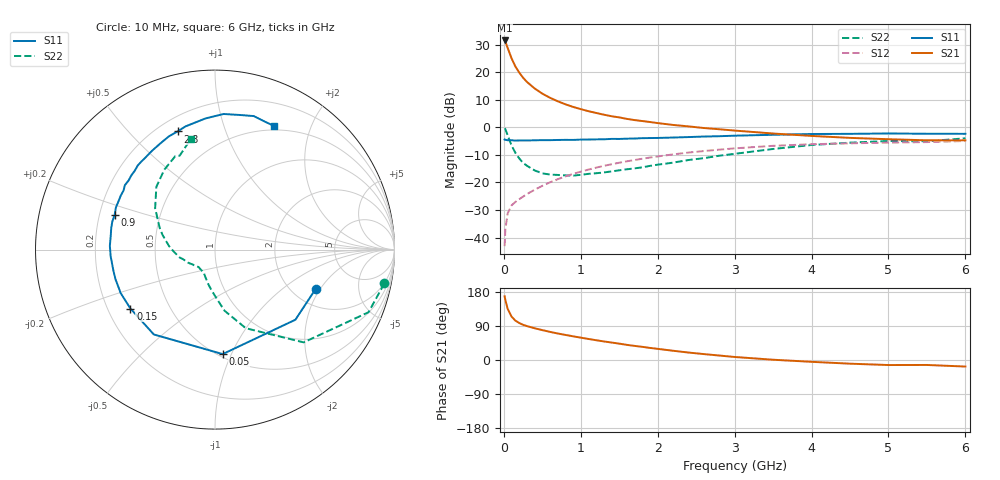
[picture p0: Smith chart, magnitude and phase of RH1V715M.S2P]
! SIEMENS Small Signal Semiconductors
! BFR106
! Si NPN RF Bipolar Junction Transistor in SOT23
! VCE = 1.75 V  IC = 15 mA
! Common Emitter S-Parameters:  August  1996
# GHz  S  MA  R  50
!  f  S11  S21  S12  S22
! GHz  MAG  ANG  MAG  ANG  MAG  ANG  MAG  ANG
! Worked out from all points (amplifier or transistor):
!   36 points, 10 MHz to 6 GHz, reference 50 ohm
!   highest |S21| = 31.5 dB at 10 MHz (marker M1)
!   |S21| within 3 dB of that: start of sweep to 53.49 MHz
!   unconditionally stable (mu >= 1): 393.3 MHz to 2.511 GHz; 4.668 GHz to end of sweep
!   at 250 MHz: K = 0.84, MSG = 21.6 dB, |S12| = -25.1 dB
!   at 1.4 GHz: K = 1.09, MAG = 6.9 dB, |S12| = -13.4 dB
!   at 6 GHz: K = 1.02, MAG = -0.8 dB, |S12| = -5.0 dB
!   S11 on the Smith chart (normalised r, x): 10 MHz: 2.65, -1.82; 50 MHz: 0.53, -0.93; 150 MHz: 0.29, -0.29; 900 MHz: 0.26, +0.16; 2.8 GHz: 0.28, +0.69; 6 GHz: 0.45, +1.49
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0.01  0.6023 -21.3  37.64 168.2  0.007 82.6  0.9624 -11.3
0.02  0.5944 -41.1  35.84 158.2  0.0143 74.7  0.9237 -22.2
0.05  0.5837 -85.8  27.46 134.7  0.0276 57.1  0.7149 -46.3
0.1  0.5829 -125.8  17.88 114.6  0.0384 48.1  0.4704 -68.6
0.15  0.5743 -145.1  12.7 103.9  0.0444 47.1  0.3449 -81.1
0.2  0.5787 -155.2  9.844 97.7  0.0497 49.0  0.2734 -88.0
0.25  0.5784 -163.2  7.937 92.8  0.0555 51.0  0.2265 -95.0
0.3  0.5781 -168.0  6.672 89.5  0.0616 53.8  0.2014 -99.9
0.4  0.5825 -176.3  5.076 83.8  0.0737 57.2  0.1657 -108.3
0.5  0.5862 178.0  4.086 78.9  0.0869 59.1  0.1465 -114.6
0.6  0.5857 172.9  3.437 74.2  0.1007 60.3  0.1392 -119.8
0.7  0.5903 168.4  2.973 70.0  0.1146 61.1  0.1371 -124.8
0.9  0.5915 161.1  2.348 62.5  0.1434 60.9  0.133 -133.3
1.1  0.6013 153.3  1.963 55.5  0.1713 59.9  0.1434 -140.5
1.3  0.6065 147.2  1.697 49.0  0.2003 58.1  0.1517 -147.7
1.6  0.6232 138.3  1.423 39.9  0.2423 54.8  0.1736 -157.5
2.2  0.6534 122.3  1.105 24.4  0.3232 46.3  0.229 -176.9
2.8  0.6904 107.6  0.924 11.8  0.3939 36.8  0.3058 163.9
3.5  0.7328 94.1  0.773 0.7  0.4621 25.7  0.4052 145.4
4.5  0.7626 79.6  0.644 -9.7  0.5134 10.5  0.5273 122.4
5.5  0.7649 68.5  0.582 -13.1  0.54 1.0  0.559 110.6
6  0.7634 64.5  0.581 -17.3  0.5655 -6.0  0.6326 102.2
